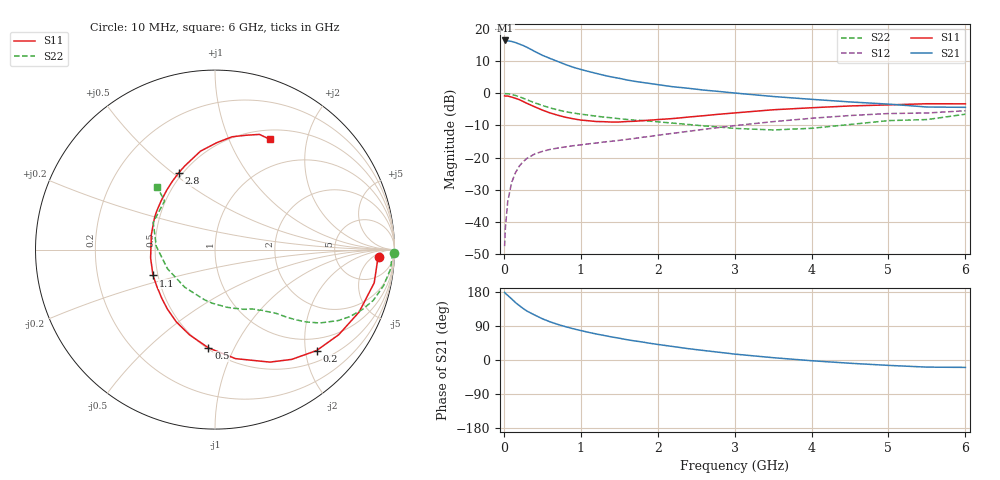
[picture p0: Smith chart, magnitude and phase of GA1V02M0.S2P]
! Infineon Technologies  Discrete & RF Semiconductors
! BF775
! Si NPN RF Bipolar Junction Transistor in SOT23
! VCE = 1 V  IC = 2 mA
! Common Emitter S-Parameters:  May  1996
# GHz  S  MA  R  50
!  f  S11  S21  S12  S22
! GHz  MAG  ANG  MAG  ANG  MAG  ANG  MAG  ANG
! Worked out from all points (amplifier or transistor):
!   36 points, 10 MHz to 6 GHz, reference 50 ohm
!   highest |S21| = 16.4 dB at 20 MHz (marker M1)
!   |S21| within 3 dB of that: start of sweep to 369.7 MHz
!   unconditionally stable (mu >= 1): 1.092 GHz to end of sweep
!   at 250 MHz: K = 0.30, MSG = 18.1 dB, |S12| = -21.3 dB
!   at 1.4 GHz: K = 1.15, MAG = 7.7 dB, |S12| = -14.9 dB
!   at 6 GHz: K = 1.06, MAG = -0.9 dB, |S12| = -5.4 dB
!   S11 on the Smith chart (normalised r, x): 10 MHz: 18, -8; 200 MHz: 0.72, -2.23; 500 MHz: 0.51, -0.80; 1.1 GHz: 0.47, -0.16; 2.8 GHz: 0.48, +0.52; 6 GHz: 0.61, +1.43
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0.01  0.9118 -2.5  6.584 178.4  0.0042 87.5  0.9957 -1.2
0.02  0.9067 -4.7  6.63 176.0  0.008 88.2  0.9869 -2.4
0.05  0.9062 -11.8  6.543 170.5  0.0205 83.0  0.9846 -6.2
0.1  0.875 -23.4  6.406 161.5  0.0405 76.0  0.9603 -12.1
0.15  0.8368 -34.5  6.159 151.7  0.058 69.7  0.9261 -17.8
0.2  0.798 -44.8  5.84 143.9  0.0735 64.7  0.8853 -22.2
0.25  0.7465 -55.0  5.537 136.1  0.0864 59.6  0.8394 -26.4
0.3  0.6975 -64.0  5.193 129.2  0.0972 55.8  0.7928 -29.9
0.4  0.6178 -79.4  4.492 118.7  0.1137 49.4  0.7129 -35.0
0.5  0.5487 -93.8  3.902 108.9  0.1248 45.3  0.647 -38.5
0.6  0.4955 -106.7  3.487 100.8  0.1341 42.2  0.5937 -41.1
0.7  0.4564 -118.3  3.128 94.0  0.1406 40.4  0.5515 -43.2
0.9  0.402 -137.5  2.544 82.6  0.1529 38.6  0.4939 -46.1
1.1  0.3742 -157.4  2.185 73.1  0.1636 37.9  0.4572 -49.3
1.4  0.3573 -179.9  1.795 60.9  0.1797 38.2  0.4156 -54.2
1.6  0.3644 167.2  1.612 53.6  0.192 39.0  0.3921 -57.6
2.2  0.4051 137.7  1.263 35.5  0.2388 39.3  0.3437 -72.1
2.8  0.4727 115.4  1.067 20.4  0.2943 36.6  0.2988 -93.2
3.5  0.5544 98.4  0.892 6.1  0.3625 30.2  0.2692 -128.8
4.5  0.6357 81.4  0.734 -8.6  0.4513 17.9  0.3276 176.9
5.5  0.688 68.9  0.612 -18.8  0.4941 3.5  0.3904 136.1
6  0.6861 63.7  0.605 -19.5  0.535 -0.4  0.473 132.7
